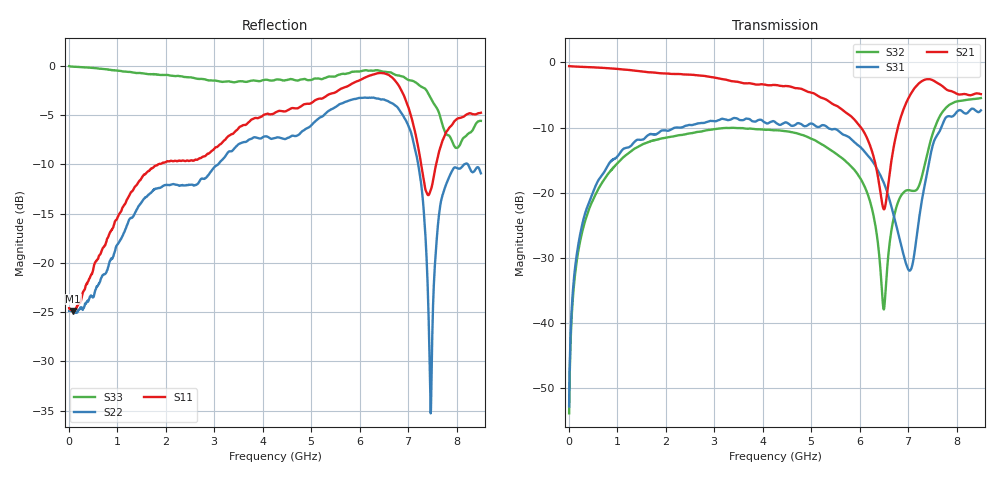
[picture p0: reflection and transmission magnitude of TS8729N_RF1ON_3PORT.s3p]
!Created with skrf (http://scikit-rf.org).
# GHz S RI R 50.0
!freq ReS11 ImS11 ReS12 ImS12 ReS13 ImS13
! ReS21 ImS21 ReS22 ImS22 ReS23 ImS23
! ReS31 ImS31 ReS32 ImS32 ReS33 ImS33
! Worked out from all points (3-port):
!   1601 points, 10 MHz to 8.5 GHz, reference 50 ohm
!   strongest paths, dB at 10 MHz, 2.132 GHz, 4.255 GHz, 6.378 GHz, 8.5 GHz:
!     S21: -0.6, -1.8, -3.4, -17.5, -4.9
!     S31: -52.9, -10.2, -9.1, -16.6, -7.4
!     S32: -53.9, -11.4, -10.4, -27.8, -5.5
!   lowest |S11| = -24.9 dB at 94.9 MHz (marker M1), VSWR 1.12, Z = 55.6 - j2.12 ohm
!   |S11| at or under -10 dB: start of sweep to 1.845 GHz; 7.268 GHz to 7.577 GHz (308.8 MHz wide, 4.16 % of centre)
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0.01  0.0589 -0.00139  0.9362 -0.00675  0.000604 0.00219
      0.9364 -0.00697  0.0571 -0.000778  0.000582 0.00194
      0.000595 0.0022  0.000569 0.00194  0.9977 -0.0116
0.0949  0.0537 -0.019  0.9307 -0.0453  0.00181 0.0189
        0.931 -0.0452  0.0551 -0.0168  0.00174 0.0167
        0.0018 0.0189  0.00174 0.0167  0.9877 -0.0894
1.745144  -0.159 -0.2604  0.6129 -0.571  0.2642 0.0925
          0.6128 -0.5709  -0.1789 -0.1506  0.2476 0.0429
          0.2644 0.0927  0.2478 0.0427  0.0429 -0.9091
4.255  -0.562 -0.1373  -0.0881 -0.6663  0.2021 -0.2848
       -0.0897 -0.6665  -0.344 0.2586  0.0737 -0.2925
       0.2012 -0.2855  0.0744 -0.2921  -0.8329 -0.1727
5.99545  -0.7419 0.4055  -0.2836 -0.1637  -0.1091 -0.1998
         -0.2839 -0.1631  0.188 0.6616  -0.1067 -0.078
         -0.1096 -0.1996  -0.1065 -0.0782  -0.6302 0.6934
6.499544  -0.5919 0.7014  -0.0227 -0.0709  -0.0978 -0.0676
          -0.0228 -0.071  0.5742 0.3568  -0.000841 -0.0126
          -0.0979 -0.0676  -0.000789 -0.0127  -0.3335 0.8741
7.035475  -0.00505 0.5841  0.1182 -0.5449  -0.0251 -0.000336
          0.1186 -0.5455  0.4049 -0.2512  0.0657 -0.0812
          -0.0252 -0.000358  0.0655 -0.0811  0.339 0.7751
7.465281  -0.133 0.193  -0.3561 -0.6492  0.1104 0.165
          -0.3569 -0.6494  0.0172 -0.000772  0.2275 -0.1086
          0.1108 0.1649  0.2281 -0.1081  0.6837 0.0954
7.709369  -0.3148 0.2751  -0.4666 -0.4618  0.3239 0.0861
          -0.4675 -0.4613  0.0403 0.2173  0.2606 -0.3264
          0.324 0.085  0.2599 -0.3266  0.3918 -0.3111
8.5  -0.3527 0.4587  -0.5026 -0.2725  0.2728 -0.3313
     -0.5023 -0.2717  0.0897 0.2705  -0.1975 -0.4945
     0.2721 -0.3315  -0.1967 -0.4952  -0.5227 -0.0623
